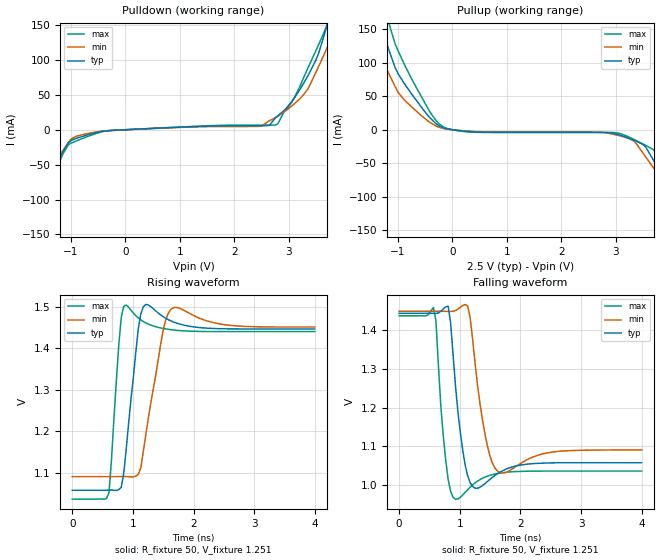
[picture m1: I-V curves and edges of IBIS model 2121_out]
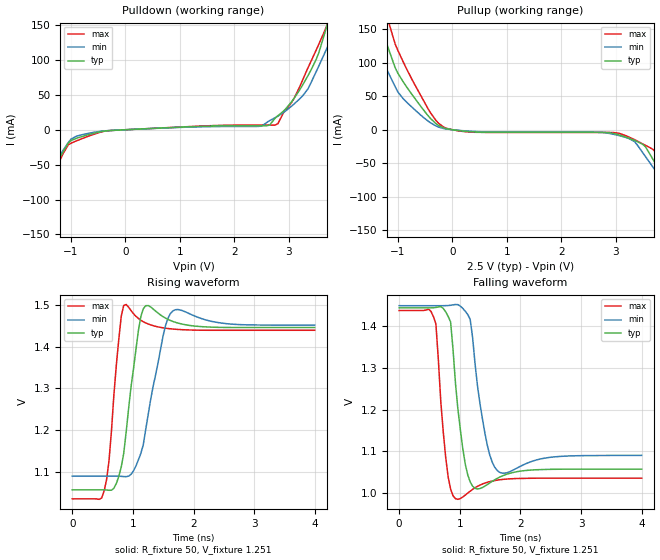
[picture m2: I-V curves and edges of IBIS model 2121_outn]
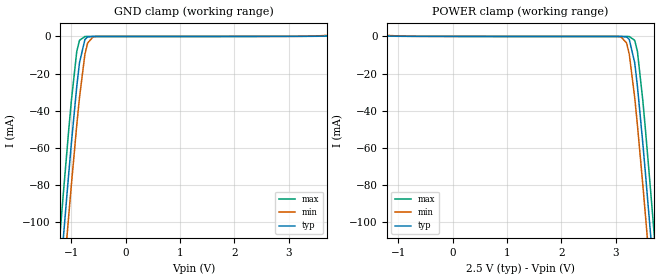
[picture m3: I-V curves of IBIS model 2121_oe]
| IBIS File eg2121l1.ibs
[IBIS ver]   3.2
[File name]   eg2121l1.ibs
[File Rev]   5
[Date]   June 23,2011
[Source]   Circiuts Simulation for EG-2121CA LVDS by HSPICE
|   Component EG-2121CA LVDS
[Component]   EG-2121L
|   (53.125M<=f<=175M, 250M<=f<=350M, 500M<=f<=700M)
[Manufacturer]   Epson Toyocom Corp.
[Package]
| variable   typ   min   max
R_pkg   1.04   NA   NA
L_pkg   1.98nH  NA   NA
C_pkg   3.71pF  NA   NA
[Pin]   signal_name   model_name   R_pin   L_pin   C_pin
1   oe   2121_oe   NA   NA   NA
4   out   2121_out   1.04   1.98n   3.71p
5   outn   2121_outn   1.04   1.98n   3.71p
6   vdd   POWER   NA   NA   NA
3   vss   GND   NA   NA   NA
[Diff Pin] inv_pin vdiff   tdelay_typ
4   5   0   0
| Models and submodels in the file (3): 2121_out (Output), 2121_outn (Output), 2121_oe (Input)
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[Model]   2121_out
Model_type Output
Enable Active-High
Polarity Non-Inverting
Vref=1.251
Vmeas=1.251
Rref=50
Cref=0
C_comp   3.84p   3.84p   3.84p
[Temperature Range] 25   85   -40
[Voltage Range]   2.5   2.35   2.65
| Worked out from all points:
|   slope of the pulldown table from 0 to 0.375 V, typ, clamps not added: 262 ohm
|   slope of the pullup table from 0 to 0.375 V, typ, clamps not added: 121 ohm
|   falling waveform, R_fixture 50, V_fixture 1.251: 20-80 % time 135ps typ, 170ps min, 104ps max; typ from 1.44 V to 1.06 V
|   rising waveform, R_fixture 50, V_fixture 1.251: 20-80 % time 159ps typ, 242ps min, 105ps max; typ from 1.06 V to 1.45 V
[Pullup]
-2.5V     451.8mA    333.9mA    593.3mA
-1.6V     223.8mA    158.6mA    300mA
-1.3V     150.9mA    106.3mA    202.6mA
-1.15V    115.4mA    80.84mA    154.9mA
-700mV    47.99mA    30.55mA    68.71mA
-150mV    2.358mA    1.587mA    3.513mA
2.75V     -3.908mA   -4.051mA   -4.037mA
3.4V      -17.81mA   -23mA      -17.04mA
3.7V      -46.24mA   -57.45mA   -30.2mA
4.45V     -145.4mA   -140.2mA   -150.7mA
4.6V      -166.2mA   -156.8mA   -178.3mA
5V        -219.5mA   -199.6mA   -249.6mA
[Pulldown]
-2.5V     -237.7mA   -199.7mA   -295.5mA
-2.05V    -172.9mA   -146.1mA   -212mA
-1.9V     -149.6mA   -127mA     -182.1mA
-1.75V    -125.8mA   -107.6mA   -151.6mA
-1.15V    -32.08mA   -29.85mA   -34.8mA
-900mV    -12.22mA   -9.263mA   -15.92mA
-300mV    -1.226mA   -1.149mA   -1.274mA
2.75V     16.63mA    17.27mA    6.689mA
3.35V     77.13mA    58.16mA    88.32mA
3.7V      148.8mA    116.7mA    149.4mA
3.95V     214.7mA    160.5mA    223.4mA
5V        506mA      371.6mA    562.4mA
[Falling Waveform]
R_fixture=50
V_fixture=1.251
V_fixture_min=1.27
V_fixture_max=1.237
0s        1.444V     1.449V     1.438V
565.7ps   1.444V     1.449V     1.459V
606.1ps   1.444V     1.449V     1.426V
808.1ps   1.463V     1.449V     1.014V
929.3ps   1.257V     1.451V     962mV
1.051ns   1.088V     1.465V     973.5mV
1.172ns   1.005V     1.432V     993.6mV
1.414ns   1.003V     1.132V     1.019V
1.616ns   1.028V     1.036V     1.029V
4ns       1.057V     1.09V      1.035V
[Rising Waveform]
R_fixture=50
V_fixture=1.251
V_fixture_min=1.27
V_fixture_max=1.237
0s        1.058V     1.091V     1.036V
606.1ps   1.058V     1.091V     1.053V
767.7ps   1.059V     1.091V     1.408V
848.5ps   1.098V     1.091V     1.5V
1.091ns   1.448V     1.096V     1.472V
1.212ns   1.505V     1.19V      1.461V
1.495ns   1.476V     1.44V      1.447V
1.657ns   1.464V     1.496V     1.444V
2.545ns   1.446V     1.456V     1.44V
4ns       1.446V     1.451V     1.44V
[Ramp]
R_load=50
dV/dt_r   2.330E-1/1.591E-10   NA   NA
dV/dt_f   2.325E-1/1.345E-10   NA   NA
|[End   2121_out
[Model]   2121_outn
Model_type Output
Enable Active-High
Polarity Inverting
Vref=1.251
Vmeas=1.251
Rref=50
Cref=0
C_comp   3.84p   3.84p   3.84p
[Temperature Range] 25   85   -40
[Voltage Range]   2.5   2.35   2.65
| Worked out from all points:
|   slope of the pulldown table from 0 to 0.375 V, typ, clamps not added: 262 ohm
|   slope of the pullup table from 0 to 0.375 V, typ, clamps not added: 121 ohm
|   falling waveform, R_fixture 50, V_fixture 1.251: 20-80 % time 150ps typ, 185ps min, 119ps max; typ from 1.44 V to 1.06 V
|   rising waveform, R_fixture 50, V_fixture 1.251: 20-80 % time 192ps typ, 272ps min, 132ps max; typ from 1.06 V to 1.45 V
[Pullup]
-2.5V     451.8mA    333.9mA    593.3mA
-1.6V     223.8mA    158.6mA    300mA
-1.3V     150.9mA    106.3mA    202.6mA
-1.15V    115.4mA    80.84mA    154.9mA
-700mV    47.99mA    30.55mA    68.71mA
-150mV    2.358mA    1.587mA    3.513mA
2.75V     -3.908mA   -4.051mA   -4.037mA
3.4V      -17.81mA   -23mA      -17.04mA
3.7V      -46.24mA   -57.45mA   -30.2mA
4.45V     -145.4mA   -140.2mA   -150.7mA
4.6V      -166.2mA   -156.8mA   -178.3mA
5V        -219.5mA   -199.6mA   -249.6mA
[Pulldown]
-2.5V     -237.7mA   -199.7mA   -295.5mA
-2.05V    -172.9mA   -146.1mA   -212mA
-1.9V     -149.6mA   -127mA     -182.1mA
-1.75V    -125.8mA   -107.6mA   -151.6mA
-1.15V    -32.08mA   -29.85mA   -34.8mA
-900mV    -12.22mA   -9.263mA   -15.92mA
-300mV    -1.226mA   -1.149mA   -1.274mA
2.75V     16.63mA    17.27mA    6.689mA
3.35V     77.13mA    58.16mA    88.32mA
3.7V      148.8mA    116.7mA    149.4mA
3.95V     214.7mA    160.5mA    223.4mA
5V        506mA      371.6mA    562.4mA
[Falling Waveform]
R_fixture=50
V_fixture=1.251
V_fixture_min=1.27
V_fixture_max=1.237
0s        1.444V     1.449V     1.438V
606.1ps   1.445V     1.449V     1.406V
767.7ps   1.435V     1.45V      1.086V
848.5ps   1.411V     1.45V      1.009V
929.3ps   1.263V     1.452V     986.1mV
1.051ns   1.106V     1.443V     990.3mV
1.172ns   1.026V     1.417V     1.004V
1.414ns   1.016V     1.144V     1.024V
1.616ns   1.035V     1.054V     1.031V
4ns       1.057V     1.09V      1.035V
[Rising Waveform]
R_fixture=50
V_fixture=1.251
V_fixture_min=1.27
V_fixture_max=1.237
0s        1.058V     1.091V     1.036V
525.3ps   1.058V     1.091V     1.055V
606.1ps   1.057V     1.091V     1.127V
686.9ps   1.062V     1.091V     1.285V
848.5ps   1.145V     1.089V     1.498V
1.091ns   1.438V     1.13V      1.467V
1.212ns   1.498V     1.203V     1.457V
1.495ns   1.472V     1.423V     1.445V
1.657ns   1.46V      1.485V     1.442V
4ns       1.446V     1.452V     1.439V
[Ramp]
R_load=50
dV/dt_r   2.328E-1/1.899E-10   NA   NA
dV/dt_f   2.323E-1/1.458E-10   NA   NA
|[End   2121_outn
[Model]   2121_oe
Model_type Input
Vinh=1.75
Vinl=0.75
C_comp   3p   3p   3p
[Temperature Range] 25   85   -40
[Voltage Range]   2.5   2.35   2.65
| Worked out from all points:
|   GND clamp passes 1 mA (typ) near -0.73 V on its own axis
|   POWER clamp passes 1 mA (typ) near -1.64 V on its own axis
[GND Clamp]
-2.5V     -614.1mA   -635.2mA   -592.4mA
-1.2V     -127.3mA   -150mA     -103.5mA
-1.15V    -109.5mA   -132.2mA   -85.68mA
-1.05V    -74.64mA   -97.23mA   -51.09mA
-1V       -57.87mA   -80.21mA   -34.8mA
-900mV    -26.94mA   -47.79mA   -8.114mA
-850mV    -14.21mA   -32.96mA   -2.138mA
-750mV    -1.674mA   -9.601mA   -76.22uA
-700mV    -312uA     -3.576mA   -59.18uA
-550mV    -37.86uA   -75.63uA   -57.57uA
3.35V     44.48uA    81.69uA    49.55uA
5V        2.629mA    2.956mA    2.308mA
[POWER Clamp]
-2.5V     2.629mA    2.956mA    2.308mA
-850mV    44.48uA    81.69uA    49.55uA
3.05V     -37.86uA   -75.63uA   -57.57uA
3.2V      -312uA     -3.576mA   -59.18uA
3.25V     -1.674mA   -9.601mA   -76.22uA
3.35V     -14.21mA   -32.96mA   -2.138mA
3.4V      -26.94mA   -47.79mA   -8.114mA
3.5V      -57.87mA   -80.21mA   -34.8mA
3.55V     -74.64mA   -97.23mA   -51.09mA
3.65V     -109.5mA   -132.2mA   -85.68mA
3.7V      -127.3mA   -150mA     -103.5mA
5V        -614.1mA   -635.2mA   -592.4mA
